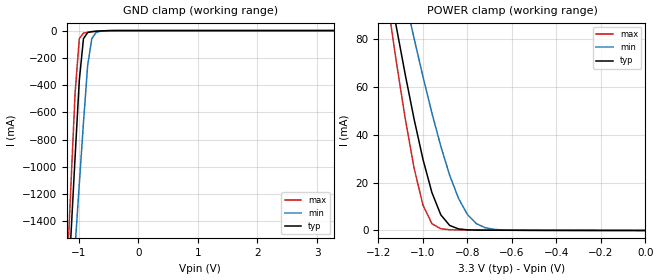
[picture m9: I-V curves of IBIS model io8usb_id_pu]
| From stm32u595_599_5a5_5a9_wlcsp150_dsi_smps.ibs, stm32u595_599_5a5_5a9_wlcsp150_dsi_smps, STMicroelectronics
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|   Model io8usb_id_pu
[Model]  io8usb_id_pu
Model_type Input
Polarity   Inverting
Vinl =   0.990000V
Vinh =   2.310000V
C_comp   2.806600pF   2.789500pF   2.832700pF
[Temperature Range]   25.000000   0.140000k   -40.000000
[Pullup Reference]   3.300000V   2.700000V   3.600000V
[Pulldown Reference]   0.0V   0.0V   0.0V
[POWER Clamp Reference]   3.300000V   2.700000V   3.600000V
[GND Clamp Reference]   0.0V   0.0V   0.0V
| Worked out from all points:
|   GND clamp passes 1 mA (typ) near -0.54 V on its own axis
|   POWER clamp passes 1 mA (typ) near -0.85 V on its own axis
[GND_clamp]
|Voltage   I(typ)   I(min)   I(max)
-3.3V     -9.738A    -9.661A    -9.429A
-1.2V     -2.082A    -2.5A      -1.818A
-1.13V    -1.502A    -2.042A    -1.132A
-1.06V    -925mA     -1.585A    -457.2mA
-990mV    -365.8mA   -1.129A    -60.2mA
-920mV    -59.59mA   -677.3mA   -18.21mA
-850mV    -14.46mA   -258.1mA   -12.36mA
-780mV    -7.59mA    -59.03mA   -8.629mA
-710mV    -4.8mA     -14.88mA   -5.493mA
-640mV    -2.824mA   -5.051mA   -3.017mA
-360mV    -19.06uA   -107.3uA   -5.16uA
3.28V     0A         7.911nA    -6.821nA
[POWER_clamp]
|Voltage   I(typ)   I(min)   I(max)
-3.28V    1.356A     1.167A     1.665A
-1.16V    106mA      131.7mA    96.07mA
-1.12V    85.24mA    114.1mA    70.63mA
-1.08V    65.3mA     96.97mA    46.88mA
-1.04V    46.57mA    80.33mA    26.08mA
-1V       29.72mA    64.29mA    10.6mA
-960mV    15.89mA    49.15mA    2.844mA
-920mV    6.559mA    35.24mA    707.1uA
-840mV    646.8uA    13.36mA    222.1uA
-760mV    155.3uA    2.862mA    172.9uA
-640mV    91uA       202.3uA    121.5uA
0V        0A         12.61nA    0A
